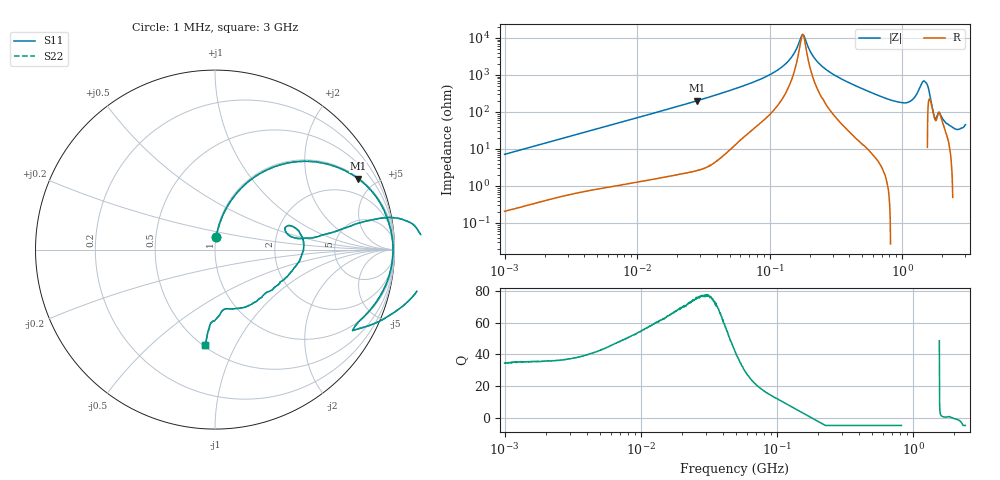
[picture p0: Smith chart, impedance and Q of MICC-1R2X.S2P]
!s-Parameter Generated by FASTRON Sdn. Bhd.
!FASTRON P/N : MICC-1R2X
!Keysight Technologies,E4991B,MY54100416,A.01.15
!Date: Fri Aug 28 09:18:54 2026
!Version  : Rev00 Fri Aug 28 09:18:54 2026
!Data & Calibration Information:
!PortZ  Port1:50+j0  Port2:50+j0
!When reading, reference impedance value at option line is always used.
! Remarks : This data is being provided solely for informational purposes.
!Freq	S11	S21	S12	S22
# Hz S dB R 50
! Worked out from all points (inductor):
!   1601 points, 1 MHz to 3 GHz, reference 50 ohm
!   read as one part in series: L = 1.14 uH near 1.041 MHz
!   highest Q = 77 at 28.29 MHz (marker M1), where L = 1.13 uH
!   self-resonance near 177.5 MHz
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1000000  -22.94 84.2  -0.04 -4.1  -0.04 -4.1  -22.94 84.2
3804036  -11.84 73.7  -0.35 -14.8  -0.35 -14.8  -11.84 73.7
1.447069e7  -3.06 44.4  -3.10 -44.7  -3.10 -44.7  -3.06 44.4
2.829425e7  -1.01 26.4  -7.04 -62.8  -7.04 -62.8  -1.01 26.4
5.477226e7  -0.30 13.3  -12.79 -75.0  -12.79 -75.0  -0.30 13.3
1.232024e8  -0.09 3.5  -24.23 -78.9  -24.23 -78.9  -0.09 3.5
1.49005e8  -0.07 1.7  -30.43 -72.9  -30.43 -72.9  -0.07 1.7
1.766402e8  -0.07 0.1  -41.78 -7.4  -41.78 -7.4  -0.07 0.1
2.083556e8  -0.07 -1.5  -31.15 71.7  -31.15 71.7  -0.07 -1.5
2.445387e8  -0.08 -3.1  -25.15 78.5  -25.15 78.5  -0.08 -3.1
3.156319e8  -0.12 -6.0  -19.58 79.6  -19.58 79.6  -0.12 -6.0
7.925923e8  -0.84 -24.7  -7.60 65.2  -7.60 65.2  -0.84 -24.7
1.054198e9  -1.01 -30.4  -5.89 62.7  -5.89 62.7  -1.01 -30.4
1.206698e9  -0.29 -25.7  -7.17 72.9  -7.17 72.9  -0.29 -25.7
1.320433e9  0.88 -15.6  -10.30 102.3  -10.30 102.3  0.88 -15.6
1.437675e9  1.41 0.2  -15.09 -178.8  -15.09 -178.8  1.41 0.2
1.557514e9  -0.37 10.7  -14.58 -72.0  -14.58 -72.0  -0.37 10.7
1.75626e9  -7.57 11.0  -4.51 -7.8  -4.51 -7.8  -7.57 11.0
1.931433e9  -6.46 -7.6  -5.47 6.8  -5.47 6.8  -6.46 -7.6
2.134733e9  -8.50 -38.8  -2.55 18.4  -2.55 18.4  -8.50 -38.8
2.581816e9  -9.49 -80.1  -0.01 19.3  -0.01 19.3  -9.49 -80.1
3e9  -5.43 -95.8  1.44 26.8  1.44 26.8  -5.43 -95.8
